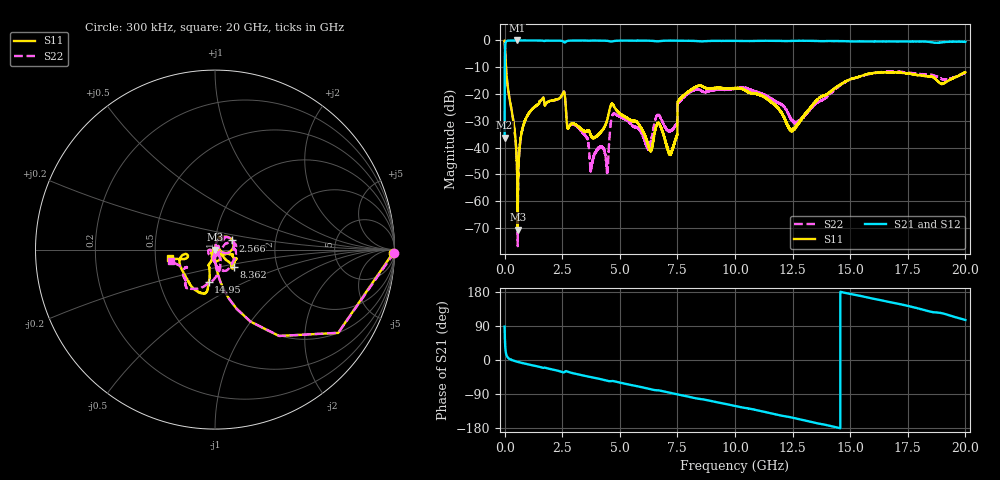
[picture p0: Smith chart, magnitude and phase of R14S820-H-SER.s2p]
!{R14S820}
!Johanson Technology Inc.
!www.johansontechnology.com
!Test Board Conditions:
!Substrate Type  RO4350B
!Substrate Thickness  20 mil
!Substrate Dk  3.66
!TL Type: GCPW
!TL Trace Width  36 mil
!TL Gap  12 mil
!Electrode orientation  Horizontal
!DUT TOPOLOGY	SERIES
!Mounting Pad LxW  26x36 mil
! Created Wed Nov 25 17:33:21 2020
! 2 Port Network Data from SP1.SP block
! freq  magS11  angS11  magS21  angS21  magS12  angS12  magS22  angS22
# khz S ma R 50
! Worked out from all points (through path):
!   20001 points, 300 kHz to 20 GHz, reference 50 ohm
!   highest |S21| = 0.00 dB at 544.3 MHz (marker M1); lowest = -36.3 dB at 300 kHz (marker M2)
!   group delay of S21, straight-line fit = 35.1 ps
!   lowest |S11| = -70.6 dB at 568.3 MHz (marker M3), VSWR 1.00, Z = 50 + j0.013 ohm
!   |S11| at or under -10 dB: 58.57 MHz to end of sweep
!   |S22| runs from -76.8 to 0.0 dB; largest |S21 - S12| = 0.018
!   S11 on the Smith chart (normalised r, x): 300 kHz: 40, -90; 2.566 GHz: 1.21, +0.13; 8.362 GHz: 1.21, -0.23; 14.95 GHz: 0.88, -0.33; 20 GHz: 0.60, -0.06
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300  0.9917 -1.1  0.01526 88.1  0.01521 88.8  0.9987 -1.0
110300  0.1709 -81.2  0.9851 8.9  0.9841 8.8  0.1715 -81.2
544300  0.003279 -103.0  0.9999 -4.5  0.9992 -4.5  0.003449 -92.3
568300  0.0002943 153.7  0.9998 -5.0  0.9992 -4.9  0.0005585 -112.7
1067300  0.04514 78.2  0.9982 -12.1  0.9978 -12.1  0.0441 77.4
2566300  0.1096 27.9  0.9401 -32.8  0.9397 -32.8  0.1116 26.4
2776300  0.02362 32.0  0.9872 -31.6  0.9879 -31.6  0.02411 27.4
3334300  0.02195 29.9  0.9964 -39.8  0.9967 -39.8  0.02017 53.6
3769300  0.01583 -36.1  0.9941 -45.1  0.9935 -45.1  0.004652 106.2
4419300  0.02927 -49.2  0.9858 -54.1  0.9867 -54.2  0.005034 103.8
4739300  0.05995 -99.7  0.9724 -55.8  0.9725 -55.9  0.04249 -136.9
6230300  0.01127 -130.9  0.9912 -75.6  0.9904 -75.6  0.009828 -123.5
6667300  0.02876 -114.3  0.9659 -80.1  0.9656 -80.1  0.04107 -100.2
7218300  0.007912 90.2  0.9916 -87.0  0.9924 -86.9  0.02081 -80.5
7600300  0.07992 -42.6  0.9862 -92.0  0.9863 -91.9  0.07306 28.0
8362300  0.1404 -42.6  0.9728 -101.8  0.9726 -101.8  0.1225 7.9
1.00003e7  0.1289 -22.7  0.9813 -121.2  0.9818 -121.3  0.126 -47.2
1.24443e7  0.02127 -76.3  0.9792 -151.7  0.9821 -151.6  0.03324 -96.7
1.33343e7  0.0595 -107.2  0.9831 -163.8  0.9849 -163.8  0.05555 -57.9
1.49513e7  0.1836 -101.0  0.9647 174.9  0.9643 174.8  0.1828 -97.3
1.66673e7  0.252 -108.6  0.9596 153.6  0.9522 153.4  0.2651 -124.8
2e7  0.2561 -168.9  0.9411 105.7  0.9407 105.9  0.2507 -165.4
